ORGANIZATION_BLOCK "Hardware Interrupt 0"
TITLE =
VERSION : 0.1


VAR_TEMP
  OB40_EV_CLASS : BYTE ;	//Bits 0-3 = 1 (Coming event), Bits 4-7 = 1 (Event class 1)
  OB40_STRT_INF : BYTE ;	//16#41 (OB 40 has started)
  OB40_PRIORITY : BYTE ;	//16 (Priority of 1 is lowest)
  OB40_OB_NUMBR : BYTE ;	//40 (Organization block 40, OB40)
  OB40_RESERVED_1 : BYTE ;	//Reserved for system
  OB40_RESERVED_2 : BYTE ;	//Reserved for system
  OB40_MDL_ADDR : WORD ;	//Base address of module initiating interrupt
  OB40_POINT_ADDR : DWORD ;	//Address of interrupt point on module
  OB40_DATE_TIME : DATE_AND_TIME ;	//Date and time OB40 started
END_VAR
BEGIN
END_ORGANIZATION_BLOCK

